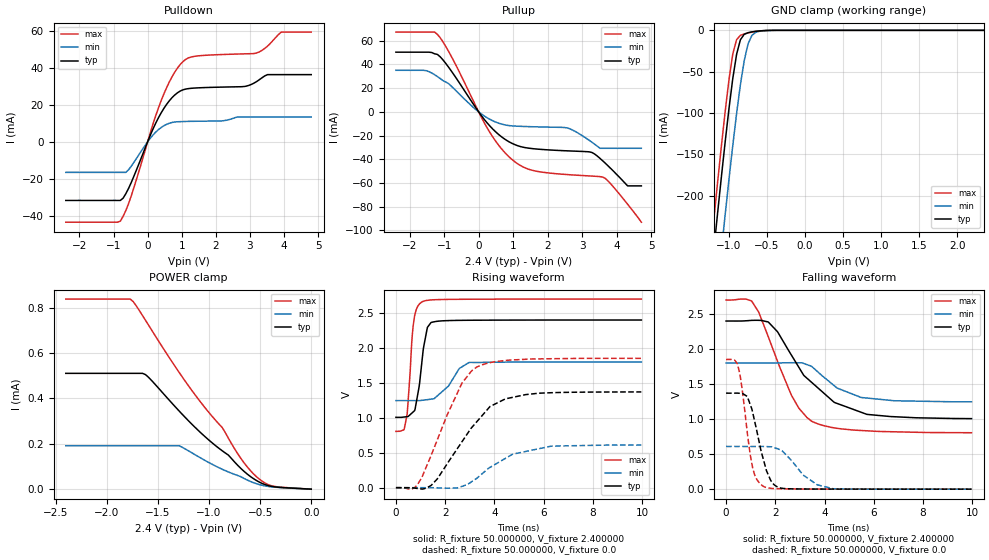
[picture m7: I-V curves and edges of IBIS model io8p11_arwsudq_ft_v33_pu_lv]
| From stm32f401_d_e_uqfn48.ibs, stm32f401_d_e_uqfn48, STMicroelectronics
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|   Model io8p11_arwsudq_ft_v33_pu_lv
[Model]  io8p11_arwsudq_ft_v33_pu_lv
Model_type I/O
Polarity   Non-Inverting
Enable   Active-Low
Vinl =   0.720000V
Vinh =   1.680000V
Vmeas =  1.200000V
Cref =   30.000000pF
Rref =   100.000000M
Vref =   0.0V
C_comp   2.828400pF   2.771400pF   2.910300pF
[Temperature Range]   25.000000   0.125000k   -40.000000
[Pullup Reference]   2.400000V   1.800000V   2.700000V
[Pulldown Reference]   0.0V   0.0V   0.0V
[POWER Clamp Reference]   2.400000V   1.800000V   2.700000V
[GND Clamp Reference]   0.0V   0.0V   0.0V
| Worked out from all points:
|   slope of the pulldown table from 0 to 0.36 V, typ, clamps not added: 25 ohm
|   slope of the pullup table from 0 to 0.36 V, typ, clamps not added: 27.7 ohm
|   GND clamp passes 1 mA (typ) near -0.62 V on its own axis
|   rising waveform, R_fixture 50.000000, V_fixture 2.400000: 20-80 % time 324ps typ, 721ps min, 218ps max; typ from 1.01 V to 2.4 V
|   rising waveform, R_fixture 50.000000, V_fixture 0.0: 20-80 % time 1.7ns typ, 1.63ns min, 1.34ns max; typ from 0.001 V to 1.37 V
|   falling waveform, R_fixture 50.000000, V_fixture 2.400000: 20-80 % time 1.94ns typ, 1.45ns min, 1.36ns max; typ from 2.4 V to 1.01 V
|   falling waveform, R_fixture 50.000000, V_fixture 0.0: 20-80 % time 554ps typ, 1.01ns min, 415ps max; typ from 1.37 V to 0.001 V
[Pulldown]
|Voltage   I(typ)   I(min)   I(max)
-2.4V     -31.66mA   -16.51mA   -43.42mA
-800mV    -31.66mA   -16.51mA   -42.86mA
-480mV    -21.98mA   -13.17mA   -29.21mA
80mV      3.63mA     1.966mA    5.014mA
480mV     18.16mA    8.738mA    26.02mA
800mV     25.38mA    10.72mA    37.77mA
1.12V     28.53mA    11.02mA    44.6mA
2.8V      29.84mA    13.46mA    47.53mA
3.2V      32.6mA     13.46mA    48.03mA
3.52V     36.33mA    13.46mA    51.75mA
3.92V     36.33mA    13.46mA    59.31mA
4.8V      36.33mA    13.46mA    59.31mA
[Pullup]
|Voltage   I(typ)   I(min)   I(max)
-2.4V     50.37mA    35.09mA    67.32mA
-1.52V    50.37mA    34.75mA    67.32mA
-1.2V     48.53mA    29.88mA    65.49mA
-800mV    34.76mA    21.92mA    47.2mA
320mV     -11.75mA   -6.207mA   -17.08mA
1.04V     -27.53mA   -11.97mA   -41.91mA
1.6V      -31.13mA   -12.57mA   -49.63mA
2.56V     -32.88mA   -13.48mA   -52.9mA
3.28V     -34.2mA    -25.51mA   -54.17mA
3.6V      -41.33mA   -30.74mA   -54.99mA
4.32V     -62.45mA   -30.74mA   -77.88mA
4.72V     -62.45mA   -30.74mA   -93.1mA
[GND_clamp]
|Voltage   I(typ)   I(min)   I(max)
-2.4V     -1.428A    -1.51A     -1.4A
-1.2V     -266.4mA   -356.3mA   -229.4mA
-1.15V    -221.3mA   -311mA     -184.1mA
-1.1V     -177.3mA   -266.4mA   -140mA
-1.05V    -134.8mA   -222.7mA   -97.97mA
-950mV    -58.22mA   -139.2mA   -28.55mA
-900mV    -29.03mA   -100.6mA   -11.27mA
-850mV    -11.41mA   -65.77mA   -6.067mA
-750mV    -2.852mA   -16.63mA   -3.179mA
-700mV    -1.914mA   -6.318mA   -2.181mA
-600mV    -750uA     -1.167mA   -738.3uA
2.35V     0A         0A         0A
[POWER_clamp]
|Voltage   I(typ)   I(min)   I(max)
-2.4V     511uA      191.4uA    838.7uA
-1.77V    511uA      191.4uA    838.7uA
-1.74V    511uA      191.4uA    826.9uA
-1.62V    505.2uA    191.4uA    744.6uA
-1.29V    344.1uA    191.4uA    514uA
-1.08V    248.7uA    137.3uA    383.1uA
-870mV    169.3uA    87.75uA    271.7uA
-720mV    105.7uA    60.5uA     157.1uA
-570mV    47.98uA    29.54uA    70.06uA
-480mV    25.17uA    16.94uA    35.08uA
-390mV    12.49uA    10.17uA    15.15uA
0V        0A         0A         0A
[Ramp]
| variable   typ   min   max
dV/dt_r  0.82171/1.70245n   0.36974/1.70203n   1.11107/1.34077n
dV/dt_f  0.83514/1.95163n   0.33174/1.45960n   1.13560/1.35735n
R_load = 50.000000
[Rising Waveform]
R_fixture= 50.000000
V_fixture= 2.400000
V_fixture_min= 1.800000
V_fixture_max= 2.700000
|time   V(typ)   V(min)   V(max)
0s        1.007V     1.247V     806mV
340.3ps   1.012V     1.247V     843mV
460.5ps   1.018V     1.247V     1.067V
700.7ps   1.085V     1.247V     2.318V
940.9ps   1.444V     1.247V     2.623V
1.061ns   1.82V      1.251V     2.659V
1.281ns   2.296V     1.261V     2.682V
1.542ns   2.374V     1.272V     2.69V
2.983ns   2.397V     1.793V     2.697V
9.97ns    2.4V       1.8V       2.7V
[Rising Waveform]
R_fixture= 50.000000
V_fixture= 0.0
V_fixture_min= 0.0
V_fixture_max= 0.0
|time   V(typ)   V(min)   V(max)
0s        957.2uV    874.7uV    1.138mV
620.6ps   -1.548mV   858.7uV    -20.43mV
860.9ps   -10.02mV   903.2uV    36.43mV
1.441ns   36.95mV    97.71uV    472.8mV
2.663ns   647.5mV    16.95mV    1.482V
3.283ns   943.8mV    134.3mV    1.727V
3.824ns   1.163V     291.9mV    1.79V
5.265ns   1.332V     518.4mV    1.838V
6.306ns   1.36V      595.2mV    1.846V
9.97ns    1.371V     610.3mV    1.852V
[Falling Waveform]
R_fixture= 50.000000
V_fixture= 2.400000
V_fixture_min= 1.800000
V_fixture_max= 2.700000
|time   V(typ)   V(min)   V(max)
0s        2.4V       1.8V       2.7V
1.041ns   2.409V     1.8V       2.685V
1.321ns   2.41V      1.8V       2.53V
1.722ns   2.384V     1.8V       2.169V
2.663ns   1.909V     1.805V     1.337V
3.163ns   1.622V     1.793V     1.073V
3.483ns   1.523V     1.751V     969mV
4.404ns   1.238V     1.474V     874.7mV
5.485ns   1.099V     1.309V     838mV
9.97ns    1.007V     1.247V     806mV
[Falling Waveform]
R_fixture= 50.000000
V_fixture= 0.0
V_fixture_min= 0.0
V_fixture_max= 0.0
|time   V(typ)   V(min)   V(max)
0s        1.371V     610.3mV    1.852V
460.5ps   1.371V     610.2mV    1.79V
660.7ps   1.367V     610.1mV    1.41V
860.9ps   1.324V     610mV      813mV
1.161ns   971.5mV    609.9mV    206mV
1.542ns   392.8mV    609.9mV    36.04mV
2.122ns   27.79mV    573.4mV    7.474mV
3.143ns   3.391mV    199.3mV    2.803mV
4.364ns   1.981mV    5.987mV    1.919mV
9.97ns    957.2uV    874.7uV    1.138mV
